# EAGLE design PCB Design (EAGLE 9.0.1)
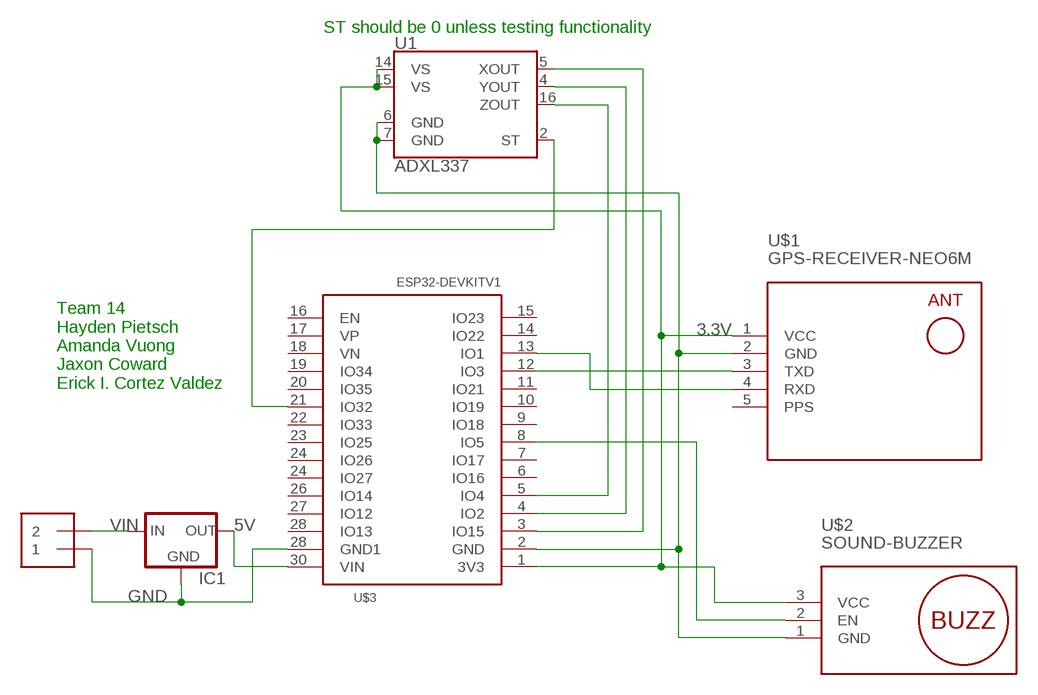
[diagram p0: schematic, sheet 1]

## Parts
IC1  V_REG_78XXSIDE  [78XXL]
J1  1X2-3.5MM  [1X2-3.5MM]
U1  ADXL337  [LFCSP-16-3X3]
U$1  GPS-RECEIVER-NEO6M  [GPS-RECEIVER-NEO6M]
U$2  SOUND-BUZZER  [SOUND-BUZZER]
U$3  ESP32DEVKITV1  [ESP32-DEVKITV1]

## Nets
3.3V [3.3V]: U1.14(VS) U1.15(VS) U$1.1(VCC) U$2.3(VCC) U$3.1(3V3)
5V [5V]: IC1.OUT U$3.30(VIN)
GND [VIN]: IC1.GND J1.1 U1.6(GND) U1.7(GND) U$1.2(GND) U$2.1(GND) U$3.2(GND) U$3.28(GND1)
N$3: U1.2(ST) U$3.21(IO32)
N$6: U1.5(XOUT) U$3.3(IO15)
N$7: U1.4(YOUT) U$3.4(IO2)
N$8: U1.16(ZOUT) U$3.5(IO4)
N$9: U$1.4(RXD) U$3.13(IO1)
N$10: U$1.3(TXD) U$3.12(IO3)
N$11: U$2.2(EN) U$3.8(IO5)
VIN [VIN]: IC1.IN J1.2
Unconnected: U$3.6(IO16) U$3.7(IO17) U$3.9(IO18) U$3.10(IO19) U$3.11(IO21) U$3.14(IO22) U$3.15(IO23) U$3.16(EN) U$3.17(VP) U$3.18(VN) U$3.19(IO34) U$3.20(IO35) U$3.22(IO33) U$3.23(IO25) U$3.24(IO26) U$3.24(IO27) U$3.26(IO14) U$3.27(IO12) U$3.28(IO13)

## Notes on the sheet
- ST should be 0 unless testing functionality
- Team 14
  Hayden Pietsch
  Amanda Vuong
  Jaxon Coward
  Erick I. Cortez Valdez

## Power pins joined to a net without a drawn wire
PPS: U$1.5(PPS)

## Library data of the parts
IC1 = SparkFun:V_REG_78XX: Voltage Regulator Standard 7805 5V regulator. IGO (Input Ground Output). Spark Fun Electronics SKU : COM-00107; MF: STMICROELECTRONICS; MPN: L7805ABV; OC_NEWARK: 34X0689
J1 = adafruit:1X2: 3.5mm Terminal block; OC_NEWARK: unknown
U1 = SparkFun-Sensors:ADXL337: Analog Devices ADXL337 3-Axis Analog Accelerometer The ADXL337 is a small, thin, low power, complete 3-axis accelerometer with signal conditioned voltage outputs. The product measures acceleration with a minimum full-scale range of ±3g. It can measure the static acceleration of gravity in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; OC_NEWARK: unknown; PROD_ID: IC-12011
U$1 = diy-modules:GPS-RECEIVER-NEO6M: GPS Receiver Module based on NEO-6 device Short tutorial how to use NEO-6 module with Arduino: http://www.xarg.org/2016/06/neo6mv2-gps-module-with-arduino/ NEO-6 datasheet is available here: https://www.u-blox.com/sites/default/files/products/documents/NEO-6_DataSheet_%28GPS.G6-HW-09005%29.pdf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; MF: NEOHM - TE CONNECTIVITY; MPN: YR1B909KCC; OC_NEWARK: 98K3962
U$2 = diy-modules:SOUND-BUZZER: Sound Buzzer Module Click here to find device on ebay.com; OC_NEWARK: unknown
U$3 = ESP32-DEVKITV1:ESP32DEVKITV1; OC_NEWARK: unknown

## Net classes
0 default: width 0.203 mm, clearance 0.127 mm
1 VIN: width 0.762 mm, clearance 0.254 mm
2 3.3V: width 0.508 mm, clearance 0.254 mm
3 5V: width 0.635 mm, clearance 0.254 mm

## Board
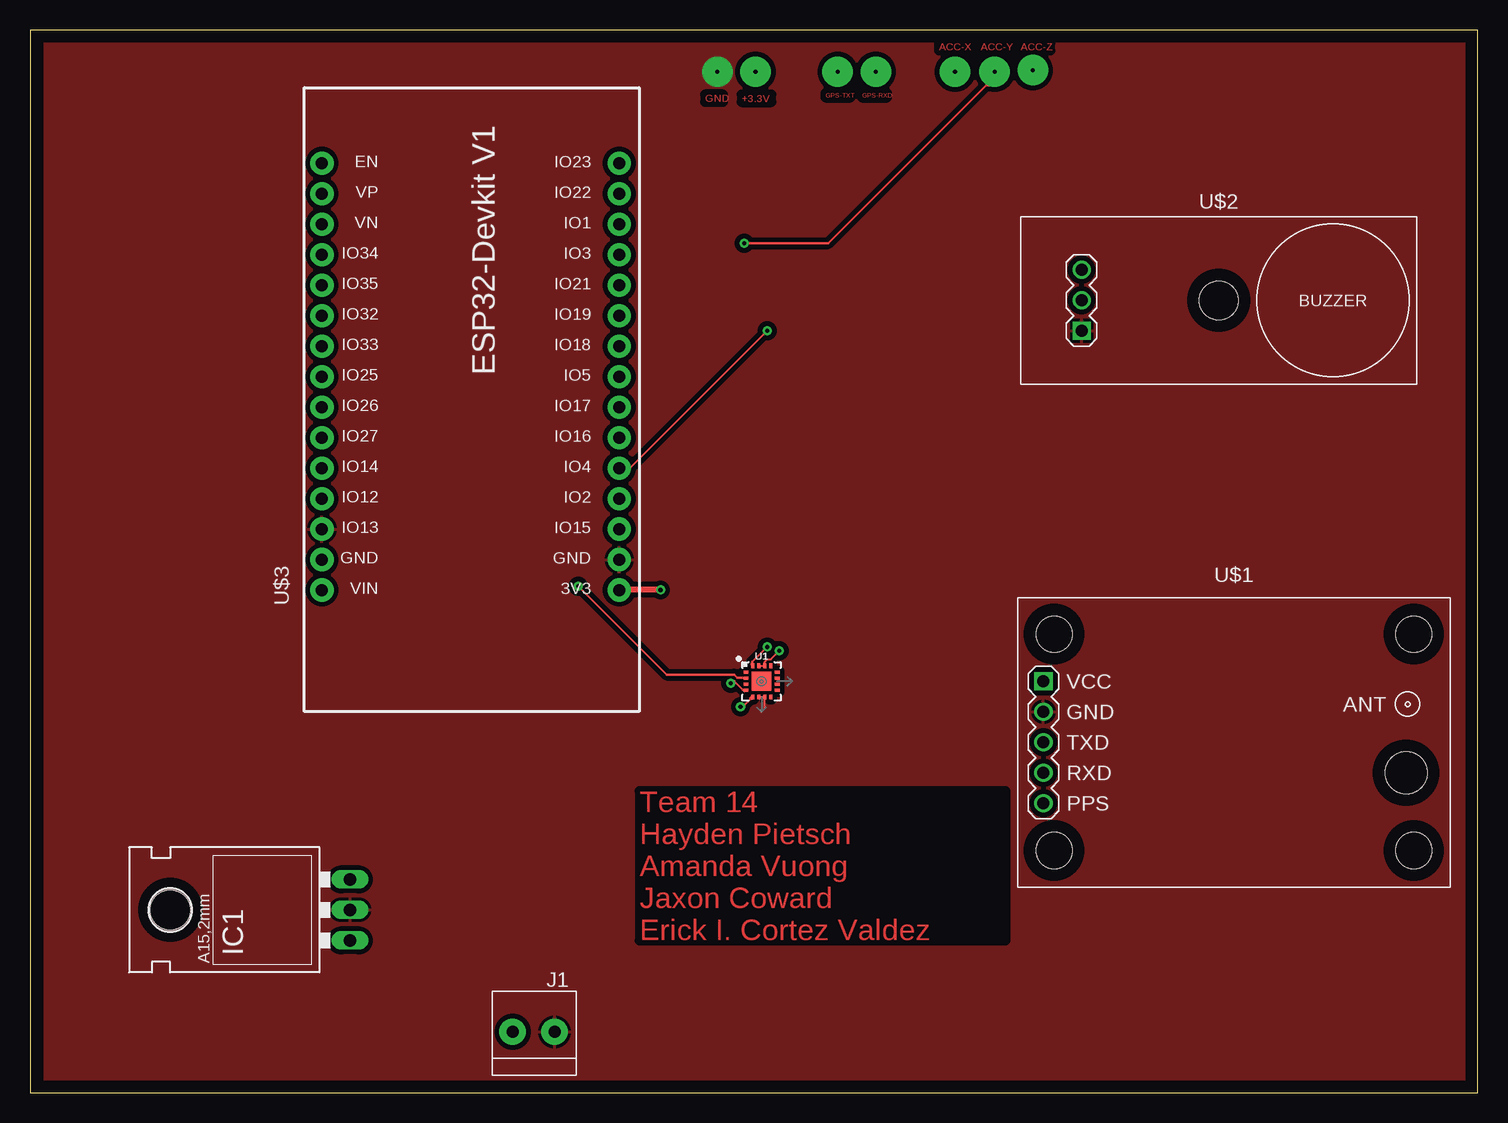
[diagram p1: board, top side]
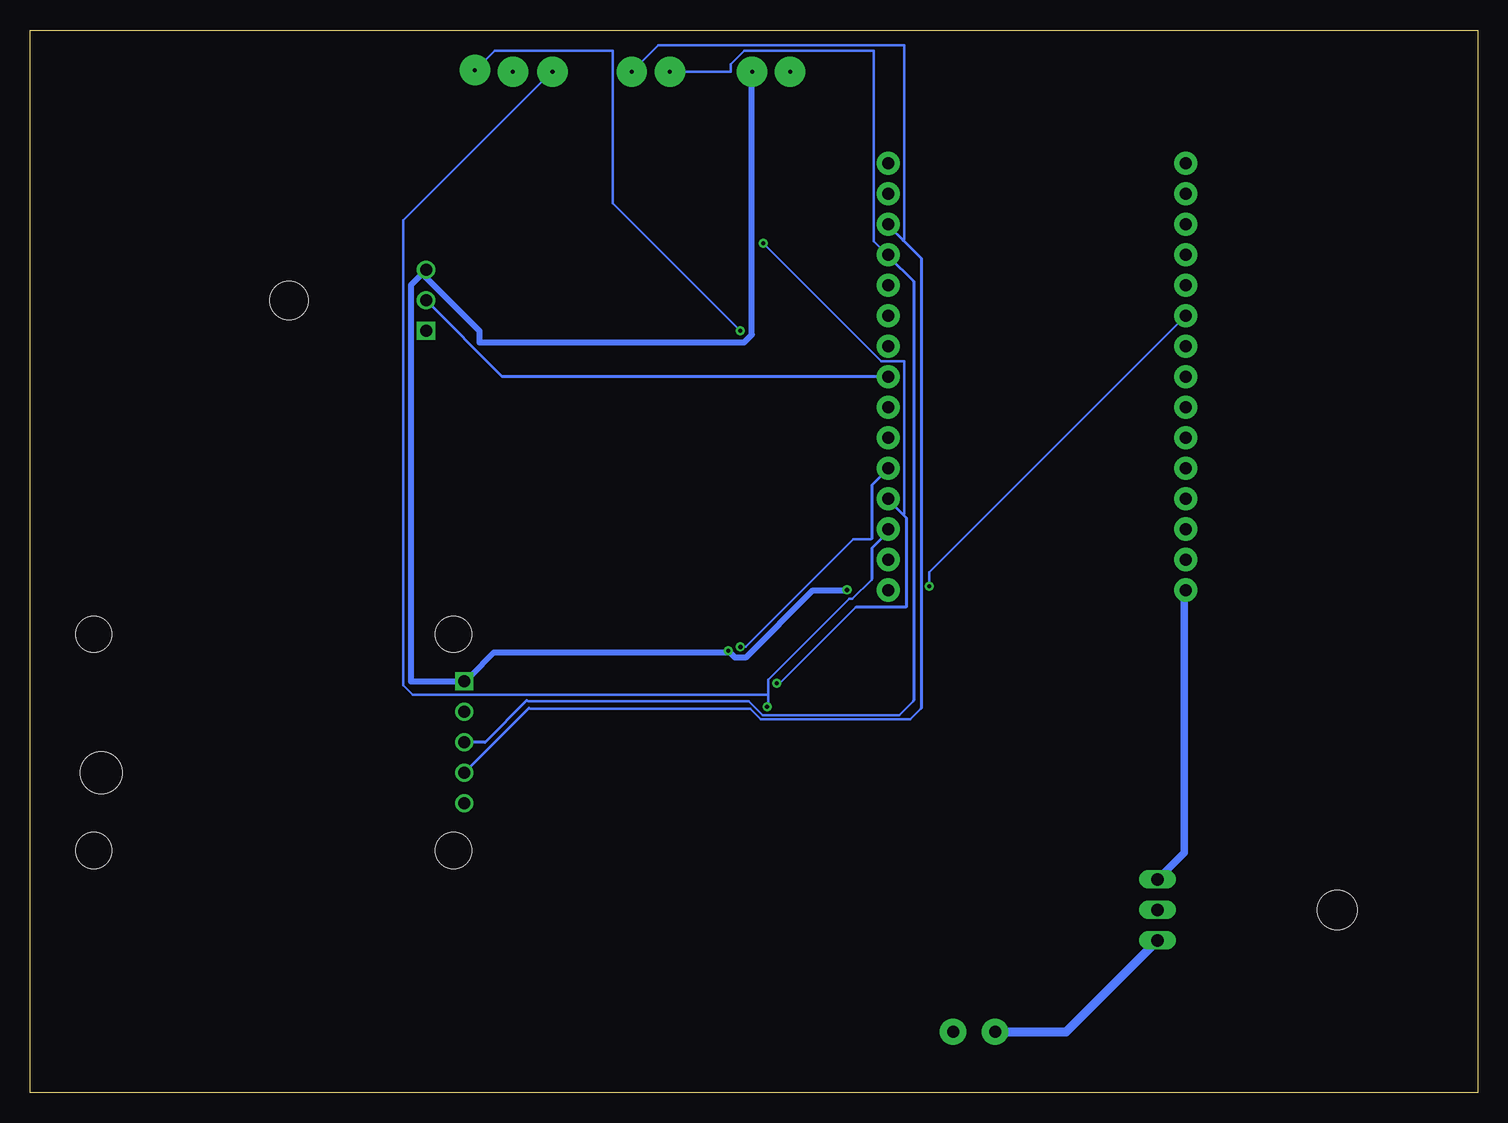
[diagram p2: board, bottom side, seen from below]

Size 120.63 x 88.57 mm. Coordinates in mm from the lower left corner, seen from the top.
Outline: 0,0 120.63,0 120.63,88.57 0,88.57 0,0
Copper layers (1*16): Top 0.035mm / dielectric 1.5mm / Bottom 0.035mm
Design rules "default": minimum track width 6mil, minimum drill 0.35mm, track to track 6mil, track to pad 6mil, pad to pad 6mil, via to via 6mil, smd to smd 6mil, copper to edge 40mil, drill to drill 6mil, minimum pad ring 10mil, minimum via ring 8mil, stop-mask expansion 4mil, vias tented up to drill 0mil, thermal gap 10mil

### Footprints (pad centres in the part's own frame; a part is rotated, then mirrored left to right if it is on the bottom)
78XXL = drill 1.016 long: GND 0,-3.81; IN -2.54,-3.81; OUT 2.54,-3.81 | hole 3.302: 0,11.176
1X2-3.5MM = drill 1 pad 2.184: 1 1.8,0; 2 -1.7,0
LFCSP-16-3X3 = smd 0.4 x 0.25: 1 -1.3,0.75; 2 -1.3,0.25; 3 -1.3,-0.25; 4 -1.3,-0.75; 9 1.3,-0.75; 10 1.3,-0.25; 11 1.3,0.25; 12 1.3,0.75 | smd 0.25 x 0.4: 5 -0.75,-1.3; 6 -0.25,-1.3; 7 0.25,-1.3; 8 0.75,-1.3; 13 0.75,1.3; 14 0.25,1.3; 15 -0.25,1.3; 16 -0.75,1.3 | smd 1.6 x 1.6: EXP 0,0
GPS-RECEIVER-NEO6M = drill 1 square: 1 -15.875,5.08 | drill 1: 2 -15.875,2.54; 3 -15.875,0; 4 -15.875,-2.54; 5 -15.875,-5.08 | hole 3: -14.986,9.017; -14.986,-9.017; 14.986,-9.017; 14.986,9.017 | hole 3.5: 14.351,-2.54
SOUND-BUZZER = drill 1 square: 1 -11.43,-2.54 | drill 1: 2 -11.43,0; 3 -11.43,2.54 | hole 3.2: 0,0
ESP32-DEVKITV1 = drill 1 pad 1.93: 1 -22.87,-13.54; 2 -20.33,-13.54; 3 -17.79,-13.54; 4 -15.25,-13.54; 5 -12.71,-13.54; 6 -10.17,-13.54; 7 -7.63,-13.54; 8 -5.09,-13.54; 9 -2.55,-13.54; 10 -0.01,-13.54; 11 2.53,-13.54; 12 5.07,-13.54; 13 7.61,-13.54; 14 10.15,-13.54; 15 12.69,-13.54; 16 12.69,11.23; 17 10.15,11.23; 18 7.61,11.23; 19 5.07,11.23; 20 2.53,11.23; 21 -0.01,11.23; 22 -2.55,11.23; 23 -5.09,11.23; 24 -7.63,11.23; 25 -10.17,11.23; 26 -12.71,11.23; 27 -15.25,11.23; 28 -17.79,11.23; 29 -20.33,11.23; 30 -22.87,11.23

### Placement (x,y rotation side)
IC1  22.86,15.24 90 top
J1  41.91,5.08 0 top
U1  60.96,34.29 0 top
U$1  100.33,29.21 0 top
U$2  99.06,66.04 0 top
U$3  35.56,64.77 90 top

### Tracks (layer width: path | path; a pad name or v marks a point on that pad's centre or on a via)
3.3V  (via drill 0.35, 0.35 pad 2.54)
  Top 0.152: v62.44,36.83 61.73,36.12 61.45,36.12 61.21,35.88 U1.14 U1.15
  Top 0.508: v52.55,41.91 49.21,41.91 U$3.1
  Bottom 0.508: U$1.1 88.9,34.29 88.9,67.31 U$2.3 87.79,68.1 83.19,63.5 83.19,62.55 61.12,62.55 60.48,63.18 60.48,85.09 v60.45,85.09 | 84.3,34.45 U$1.1 | v52.55,41.91 52.63,41.87 55.38,41.87 60.98,36.27 61.87,36.27 62.41,36.8 v62.44,36.83 62.67,36.72 81.97,36.72 83.92,34.76 U$1.1 | 84.1,34.58 U$1.1
5V
  Bottom 0.635: IC1.OUT 24.45,20 24.45,41.75 U$3.30
GND  (via drill 0.35 pad 2.54)
  Top 0.152: 60.96,31.75 61.21,32 U1.7 U1.6
  other vias: 57.28,85.09
  pour Top (isolate 0.406): 1.27,0 1.27,87.63 120.65,87.63 120.65,0
N$3  (via drill 0.35)
  Top 0.203: v45.7,42.23 53.07,34.85 58.67,34.85 58.94,34.58 59.65,34.58 U1.2
  Bottom 0.203: v45.7,42.23 45.7,43.38 24.36,64.72 U$3.21
N$6  (via drill 0.35, 0.35 pad 2.54)
  Top 0.203: 59.37,32.07 59.38,32.18 60.01,32.8 60.01,32.89 60.1,32.98 U1.5 | v59.21,32.18 59.21,32.07
  Top 0.254: 59.05,32.07 59.21,32.07 59.37,32.07 | 60.17,32.86 U1.5
  Bottom 0.203: v59.21,32.18 59.12,32.18 59.12,33.18 | 59.12,33.18 59.12,34.4 52.36,41.16 52.09,41.16 50.49,42.76 50.48,42.86 | 59.12,33.18 88.74,33.18 89.53,33.97 89.53,72.71 77.15,85.09 v77.09,85.09
  Bottom 0.254: 50.48,42.86 50.48,45.4 49.21,46.67 49.21,46.83 U$3.3
N$7  (via drill 0.35, 0.35 pad 2.54)
  Top 0.203: v58.41,34.14 58.59,34.31 58.67,34.31 59.38,33.6 59.47,33.6 U1.4 | v59.53,70.8 66.52,70.8 79.69,83.98 80.33,83.98 80.33,85.09 v80.39,85.09
  Top 0.254: 59.53,33.5 U1.4
  Bottom 0.203: v58.41,34.14 58.14,34.14 51.83,40.45 51.75,40.48 | v59.53,70.8 49.69,60.96 47.78,60.96 47.78,48.26 47.86,48.18
  Bottom 0.254: 51.75,40.48 47.62,40.48 47.62,47.94 47.86,48.18 49.05,49.37 U$3.4
N$8  (via drill 0.35, 0.35 pad 2.54)
  Top 0.203: v61.43,37.16 60.19,35.92 60.19,35.83 60.17,35.72 | v61.44,63.5 50.01,52.07 49.21,52.07 U$3.5
  Top 0.254: 60.17,35.72 U1.16
  Bottom 0.203: v61.43,37.16 60.98,37.16 52.01,46.14 50.58,46.14 50.48,46.2 | v61.44,63.5 72.07,74.14 72.07,86.84 81.92,86.84 83.5,85.25 v83.57,85.22
  Bottom 0.254: 50.48,46.2 50.48,50.64 49.21,51.91 U$3.5
N$9  (via drill 0.35 pad 2.54)
  Bottom 0.203: 79.06,32.07 78.94,32 60.63,32 59.74,31.11 47.3,31.11 46.41,32 46.35,32.07 | v70.48,85.09 68.26,87.31 47.78,87.31 47.78,71.12 47.86,71.04
  Bottom 0.254: 79.06,32.07 U$1.4 | 46.35,32.07 46.35,69.53 47.86,71.04 49.05,72.23 U$3.13
N$10  (via drill 0.35 pad 2.54)
  Bottom 0.203: 79.22,32.7 79.12,32.63 60.72,32.63 59.56,31.47 48.18,31.47 47.03,32.63 46.99,32.7 | v67.31,85.09 62.23,85.09 62.23,85.72 61.12,86.84 50.32,86.84 50.32,70.96 49.21,69.85 U$3.12
  Bottom 0.254: U$1.3 82.71,29.21 79.22,32.7 | 46.99,32.7 46.99,67.63 49.05,69.69 U$3.12
N$11
  Bottom 0.254: U$2.2 81.28,59.69 49.21,59.69 U$3.8
VIN
  Bottom 0.762: IC1.IN 34.29,5.08 J1.2

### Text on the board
Top: ACC-X | ACC-Y | ACC-Z | GND | +3.3V | GPS-TXT | GPS-RXD | Team 14 / Hayden Pietsch / Amanda Vuong / Jaxon Coward / Erick I. Cortez Valdez

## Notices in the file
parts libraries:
diy-modules: Released under the Creative Commons Attribution 4.0 International License: http://creativecommons.org/licenses/by/4.0
SparkFun-Sensors: Licensing: Creative Commons ShareAlike 4.0 International - https://creativecommons.org/licenses/by-sa/4.0
